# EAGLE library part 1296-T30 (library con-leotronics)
1.27mm SINGLE ROW FEMALE SOCKET Source: http://www.leotronics.co.uk/Conexcon/Data%20Sheets/sec.%20A/1296ing.pdf
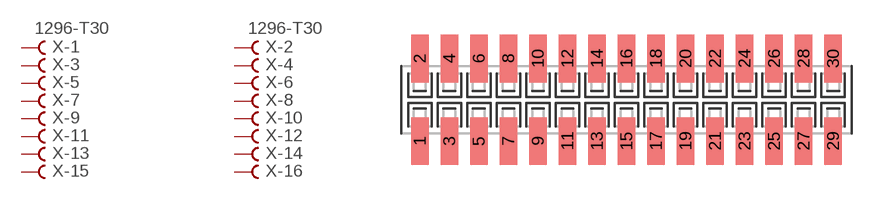
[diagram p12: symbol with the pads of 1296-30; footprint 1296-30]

Designator prefix X; gates -1=FVAL -2=FVAL -3=F -4=F -5=F -6=F -7=F -8=F -9=F -10=F -11=F -12=F -13=F -14=F -15=F -16=F -17=F -18=F -19=F -20=F -21=F -22=F -23=F -24=F -25=F -26=F -27=F -28=F -29=F -30=F

## 1296-T30 (OC_FARNELL: unknown; OC_NEWARK: unknown)  [1296-30]
1  -1:B  pas
2  -2:B  pas
3  -3:B  pas
4  -4:B  pas
5  -5:B  pas
6  -6:B  pas
7  -7:B  pas
8  -8:B  pas
9  -9:B  pas
10  -10:B  pas
11  -11:B  pas
12  -12:B  pas
13  -13:B  pas
14  -14:B  pas
15  -15:B  pas
16  -16:B  pas
17  -17:B  pas
18  -18:B  pas
19  -19:B  pas
20  -20:B  pas
21  -21:B  pas
22  -22:B  pas
23  -23:B  pas
24  -24:B  pas
25  -25:B  pas
26  -26:B  pas
27  -27:B  pas
28  -28:B  pas
29  -29:B  pas
30  -30:B  pas

## Footprint 1296-30 (pad centres in mm)
1.27mm SINGLE ROW FEMALE SOCKET Source: http://www.leotronics.co.uk/Conexcon/Data%20Sheets/sec.%20A/1296ing.pdf
smd 0.76 x 2.05: 1 -8.89,-1.78; 2 -8.89,1.78; 3 -7.62,-1.78; 4 -7.62,1.78; 5 -6.35,-1.78; 6 -6.35,1.78; 7 -5.08,-1.78; 8 -5.08,1.78; 9 -3.81,-1.78; 10 -3.81,1.78; 11 -2.54,-1.78; 12 -2.54,1.78; 13 -1.27,-1.78; 14 -1.27,1.78; 15 0,-1.78; 16 0,1.78; 17 1.27,-1.78; 18 1.27,1.78; 19 2.54,-1.78; 20 2.54,1.78; 21 3.81,-1.78; 22 3.81,1.78; 23 5.08,-1.78; 24 5.08,1.78; 25 6.35,-1.78; 26 6.35,1.78; 27 7.62,-1.78; 28 7.62,1.78; 29 8.89,-1.78; 30 8.89,1.78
